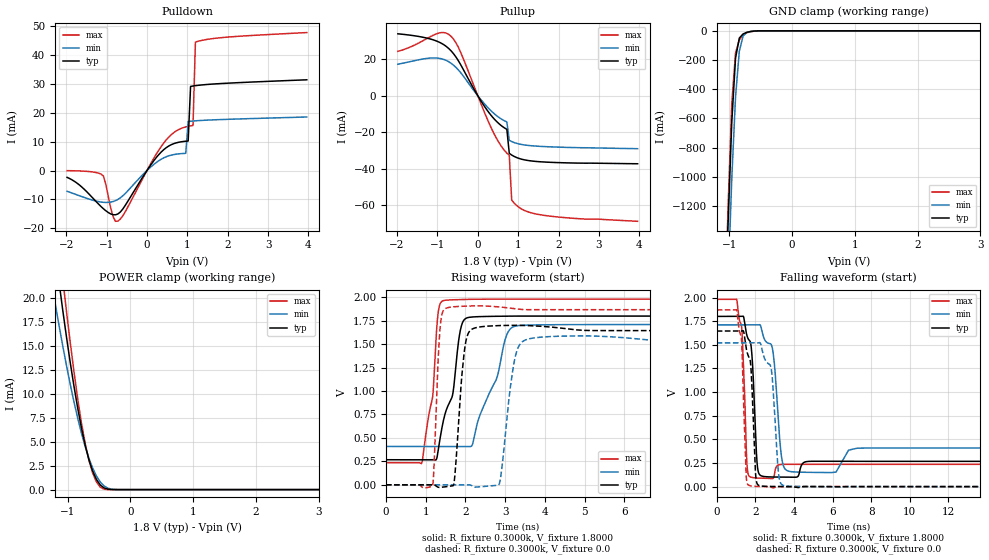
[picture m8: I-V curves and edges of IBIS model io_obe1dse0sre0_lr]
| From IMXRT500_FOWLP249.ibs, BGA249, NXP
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[Model] io_obe1dse0sre0_lr
|   Model io_obe1dse0sre0_lr
| Library cells for typ/min/max conditions are connected as defined below:
|  pad - External Pad
|  ipp_do - Core Input
|  ipp_obe - Output Buffer Enable
|  REFH3V3 - vdd1v8
|  gnde - gnde
|  ipp_ina235_3v - NC
|  ipp_ina40_3v - NC
|  ipp_ina_mux - NC
|  ipp_ind - NC
|  ipp_ind_1p8v - NC
|  ipp_ind_3v - NC
|  vdd - vdd
|  vdd1v8 - vdd1v8
|  vdda - vdde3v3
|  vdde3v3 - vdde3v3
| All other pins connected to ground
Model_type I/O
Polarity   Non-Inverting
Enable   Active-High
Vinl =   0.5400V
Vinh =   1.2600V
Vmeas =  0.9000V
Cref =   25.0000pF
Rref =   0.5000k
Vref =   0.0V
C_comp   2.2673pF   2.1740pF   2.3940pF
[Temperature Range]   25.0000   0.1250k   -40.0000
[Voltage Range]   1.8000V   1.7100V   1.9800V
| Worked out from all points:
|   slope of the pulldown table from 0 to 0.27 V, typ, clamps not added: 52.5 ohm
|   slope of the pullup table from 0 to 0.27 V, typ, clamps not added: 29.8 ohm
|   GND clamp passes 1 mA (typ) near -0.57 V on its own axis
|   POWER clamp passes 1 mA (typ) near -0.54 V on its own axis
|   rising waveform, R_fixture 0.3000k, V_fixture 1.8000: 20-80 % time 421ps typ, 635ps min, 252ps max; typ from 0.267 V to 1.8 V
|   rising waveform, R_fixture 0.3000k, V_fixture 0.0: 20-80 % time 168ps typ, 239ps min, 107ps max; typ from 0 V to 1.65 V
|   falling waveform, R_fixture 0.3000k, V_fixture 1.8000: 20-80 % time 232ps typ, 310ps min, 192ps max; typ from 1.8 V to 0.267 V
|   falling waveform, R_fixture 0.3000k, V_fixture 0.0: 20-80 % time 219ps typ, 292ps min, 174ps max; typ from 1.65 V to 0 V
[Pulldown]
|Voltage   I(typ)   I(min)   I(max)
-1.98V    -2.37mA    -7.2mA     -50uA
-1.08V    -13.25mA   -11.03mA   -1.913mA
-840mV    -15.32mA   -10.75mA   -15.99mA
-720mV    -15.07mA   -10.02mA   -17.56mA
300mV     5.63mA     3.457mA    7.23mA
600mV     8.94mA     5.324mA    12.39mA
960mV     10.15mA    5.952mA    15.11mA
1.02V     10.23mA    16.97mA    15.31mA
1.08V     29.14mA    17.07mA    15.48mA
1.14V     29.29mA    17.15mA    15.61mA
1.2V      29.41mA    17.22mA    44.52mA
3.96V     31.44mA    18.55mA    47.81mA
[Pullup]
|Voltage   I(typ)   I(min)   I(max)
-1.98V    34mA       17.32mA    24.37mA
-960mV    29.45mA    20.56mA    34.44mA
-600mV    23.04mA    16.76mA    31.06mA
-420mV    16.88mA    12.58mA    23.61mA
180mV     -6.31mA    -4.805mA   -9.918mA
480mV     -14.43mA   -11.18mA   -24.06mA
720mV     -18.43mA   -14.35mA   -31.5mA
780mV     -31.62mA   -24.45mA   -32.76mA
840mV     -32.54mA   -25.13mA   -57.28mA
1.02V     -34.39mA   -26.46mA   -61.25mA
1.8V      -36.53mA   -28.04mA   -66.1mA
3.96V     -37.33mA   -29.06mA   -68.91mA
[GND_clamp]
|Voltage   I(typ)   I(min)   I(max)
-1.98V    -17.54A    -17.55A    -18.13A
-1.08V    -2.178A    -2.567A    -2.121A
-1.02V    -1.334A    -1.74A     -1.223A
-960mV    -626.1mA   -1.012A    -499.4mA
-900mV    -186.7mA   -452.2mA   -152mA
-840mV    -49.63mA   -139.9mA   -62.86mA
-780mV    -21.48mA   -35.54mA   -26.58mA
-720mV    -10.4mA    -11.15mA   -13.18mA
-600mV    -1.573mA   -2.152mA   -2.249mA
-480mV    -123.2uA   -243.9uA   -63.17uA
3.96V     0A         0A         0A
[POWER_clamp]
|Voltage   I(typ)   I(min)   I(max)
-1.98V    72.06mA    51.35mA    77.71mA
-1.26V    28.12mA    21.78mA    33.04mA
-1.2V     24.9mA     19.47mA    29.3mA
-1.14V    21.8mA     17.23mA    25.64mA
-1.08V    18.82mA    15.06mA    22.09mA
-1.02V    15.98mA    12.99mA    18.67mA
-840mV    8.51mA     7.462mA    9.493mA
-720mV    4.608mA    4.475mA    4.783mA
-600mV    1.908mA    2.218mA    1.702mA
-540mV    1.04mA     1.402mA    786.7uA
-420mV    173.6uA    383.7uA    43.39uA
3.96V     0A         0A         0A
[Ramp]
| variable   typ   min   max
dV/dt_r  0.5848/0.1845n   0.4709/0.2716n   0.8358/0.1289n
dV/dt_f  0.7353/0.3229n   0.4996/0.4273n   0.7443/0.2287n
R_load = 50.0000
[Rising Waveform]
R_fixture= 0.3000k
V_fixture= 1.8000
V_fixture_min= 1.7100
V_fixture_max= 1.9800
|time   V(typ)   V(min)   V(max)
0s        267.3mV    408.9mV    235.9mV
901.8ps   267.3mV    408.9mV    230.6mV
1.179ns   267.6mV    408.9mV    950.9mV
1.268ns   268.6mV    408.9mV    1.604V
1.383ns   545.4mV    408.9mV    1.946V
1.898ns   1.694V     408.9mV    1.976V
2.288ns   1.793V     638.7mV    1.98V
3.142ns   1.8V       1.668V     1.981V
4.676ns   1.8V       1.71V      1.98V
500ns     1.8V       1.71V      1.98V
[Rising Waveform]
R_fixture= 0.3000k
V_fixture= 0.0
V_fixture_min= 0.0
V_fixture_max= 0.0
|time   V(typ)   V(min)   V(max)
0s        30.08nV    1.925uV    117.4nV
1.173ns   440.5uV    1.915uV    -10.38mV
1.378ns   -27.31mV   1.839uV    1.735V
1.698ns   -7.737mV   1.348uV    1.899V
1.975ns   1.43V      -10.87uV   1.905V
2.215ns   1.67V      -21.68mV   1.909V
2.853ns   1.699V     11.03mV    1.897V
3.393ns   1.701V     1.51V      1.871V
4.993ns   1.647V     1.589V     1.868V
500ns     1.645V     1.52V      1.868V
[Falling Waveform]
R_fixture= 0.3000k
V_fixture= 1.8000
V_fixture_min= 1.7100
V_fixture_max= 1.9800
|time   V(typ)   V(min)   V(max)
0s        1.8V       1.71V      1.98V
1.036ns   1.8V       1.71V      1.981V
1.393ns   1.795V     1.71V      1.246V
1.625ns   1.565V     1.71V      136.6mV
1.826ns   1.389V     1.71V      97.13mV
2.131ns   179.8mV    1.709V     90.73mV
2.882ns   101.8mV    1.465V     84.31mV
3.477ns   100.1mV    209.1mV    235.5mV
5.73ns    268mV      148.7mV    236mV
500ns     267.3mV    408.9mV    235.9mV
[Falling Waveform]
R_fixture= 0.3000k
V_fixture= 0.0
V_fixture_min= 0.0
V_fixture_max= 0.0
|time   V(typ)   V(min)   V(max)
0s        1.645V     1.52V      1.868V
1.048ns   1.645V     1.52V      1.859V
1.292ns   1.645V     1.52V      1.533V
1.58ns    1.417V     1.52V      34.9mV
1.775ns   1.256V     1.52V      7.307mV
2.056ns   58.05mV    1.519V     2.63mV
2.939ns   1.596mV    976.8mV    -13.08mV
3.33ns    1.069mV    31.66mV    581.4uV
6.115ns   348uV      -5.876mV   18.74uV
500ns     1.042uV    3.179uV    680.8nV
